FUNCTION_BLOCK FB_IEDClient IMPLEMENTS I_ScsmAbortIndEventSink, I_ScsmGetServerDirectoryCnfEventSink, I_ScsmGetLogicalDeviceDirectoryCnfEventSink, I_ScsmGetLogicalNodeDirectoryCnfEventSink, I_ScsmGetDataValuesCnfEventSink, I_ScsmSetDataValuesCnfEventSink, I_ScsmReportIndEventSink, I_ScsmControlCnfEventSink, I_ScsmLastApplErrorIndEventSink, I_ScsmCommandTerminationIndEventSink
VAR_INPUT
	fbConnection		: FB_iec61850ClientClass := (ipAbortInd:=THIS^, ipGetServerDirectoryCnf:=THIS^, ipGetLogicalDeviceDirectoryCnf:=THIS^, ipGetLogicalNodeDirectoryCnf:=THIS^, ipGetDataValuesCnf:=THIS^, ipSetDataValuesCnf:=THIS^, ipReportInd:=THIS^, ipControlCnf:=THIS^, ipLastApplErrorInd:=THIS^, ipCommandTerminationInd:=THIS^);
END_VAR
VAR
	_bAbort				: BOOL; (* Rising edge activates AbortReq() command execution *)
	_bDisconnect		: BOOL; (* Rising edge activates ReleaseReq() command execution *)
	_bConnect			: BOOL; (* Rising edge activates AssociateReq() command execution *)
	_bReconnect			: BOOL := TRUE; (* TRUE => reconnect automatically *)
	_bReadAllData		: BOOL := TRUE; (* TRUE => read/refresh all data values on reconnect *)
	
	state				: BYTE;
	eState				: E_AsyncEnvironmentState; (* Environment state *)
	bBusy				: BOOL; (* If TRUE => command execution is busy *)
	bSuccess			: BOOL;
	ipResult			: I_AsyncServiceResultClass;
	sLastErrorResult	: T_MaxString;
	fbAbortReason		: FB_ServiceErrorClass := (stError:=SUCCESS_EVENT);
	sLastAbortReason	: T_MaxString;
	nInvokeID			: UDINT;
	eServiceError		: E_AcsiServiceError; (* Latest OnXyzCnf() or OnXyzInd() event handler error *)
	nServiceError		: UDINT; (* Counts OnXyzCnf() and OnXyzInd() event handler errors *)
	nCmdError			: UDINT; (* Counts xyzReq() command errors *)
	sObjReference		: T_AcsiObjectReference; (* DATA object reference *)
	sCtrlReference		: T_AcsiObjectReference; (* CONTROLLABLE-DATA object reference *)

	bGetServerDirectory				: BOOL := TRUE; (* Rising edge enumerates logical-devices *)
	bGetLogicalDeviceDirectory		: BOOL := TRUE; (* Rising edge enumerates logical-nodes *)
	bGetLogicalNodeDirectory		: BOOL := TRUE; (* Rising edge enumerates "IEDLD1/LLN0" data-sets *)
	bGetAllServerValues				: BOOL := TRUE; (* Rising edge reads all "IEDLD1" data attribute values *)
	bGetAllDataValues_LLN0_ST		: BOOL := TRUE; (* Rising edge reads all "IEDLD1/LLN0.ST" data attribute values (having selected functional constraint) *)
	bGetDataValues_LLN0_ST_Beh		: BOOL := TRUE; (* Rising edge reads all "IEDLD1/LLN0.ST.Beh" data attribute values (having selected functional constraint) *)

	(* Low-Level/basic control of reporting using single commands to read/write RCB data attribute values *)
	bGetUrCBValues_urcb101			: BOOL := TRUE; (* Rising edge reads all "IEDLD1/LLN0.urcb101" data attribute values *)
	bGetUrCBValues_urcb201			: BOOL := TRUE; (* Rising edge reads all "IEDLD1/LLN0.urcb201" data attribute values *)
	bGetUrCBValues_urcb301			: BOOL := TRUE; (* Rising edge reads all "IEDLD1/LLN0.urcb301" data attribute values *)
	bGetBrCBValues_brcb101			: BOOL := TRUE; (* Rising edge reads all "IEDLD1/LLN0.brcb101" data attribute values *)
	bGetBrCBValues_brcb201			: BOOL := TRUE; (* Rising edge reads all "IEDLD1/LLN0.brcb201" data attribute values *)
	bGetBrCBValues_brcb301			: BOOL := TRUE; (* Rising edge reads all "IEDLD1/LLN0.brcb301" data attribute values *)

	eSetUrCBValues_urcb101_Resv		: E_CtlBool := E_CtlBool.None; (* Writes True|False to "IEDLD1/LLN0.urcb101.Resv" data attribute value *)
	eSetUrCBValues_urcb101_RptEna	: E_CtlBool := E_CtlBool.None; (* Writes True|False to "IEDLD1/LLN0.urcb101.RptEna" data attribute value *)
	bSetUrCBValues_urcb101_RptID	: BOOL := FALSE; (* Rising edge writes "IEDLD1/LLN0.urcb101.RptID" data attribute value *)
	bSetUrCBValues_urcb101_TrgOps	: BOOL := FALSE; (* Rising edge writes "IEDLD1/LLN0.urcb101.TrgOps" data attribute value *)
	bSetUrCBValues_urcb101_OptFlds	: BOOL := FALSE; (* Rising edge writes "IEDLD1/LLN0.urcb101.OptFlds" data attribute value *)
	bSetUrCBValues_urcb101_IntgPd	: BOOL := FALSE; (* Rising edge writes "IEDLD1/LLN0.urcb101.IntgPd" data attribute value *)
	bSetUrCBValues_urcb101_BufTm	: BOOL := FALSE; (* Rising edge writes "IEDLD1/LLN0.urcb101.BufTm" data attribute value *)
	bSetUrCBValues_urcb101_All		: BOOL := FALSE; (* Rising edge writes multiple "IEDLD1/LLN0.urcb101" data attribute values: "RptID", "TrgOps", "OptFlds, "IntgPd" and "BufTm" *)

	eSetBrCBValues_brcb101_RptEna	: E_CtlBool := E_CtlBool.None; (* Writes True|False to "IEDLD1/LLN0.brcb101.RptEna" data attribute value *)
	bSetBrCBValues_brcb101_RptID	: BOOL := FALSE; (* Rising edge writes "IEDLD1/LLN0.brcb101.RptID" data attribute value *)
	bSetBrCBValues_brcb101_TrgOps	: BOOL := FALSE; (* Rising edge writes "IEDLD1/LLN0.brcb101.TrgOps" data attribute value *)
	bSetBrCBValues_brcb101_OptFlds	: BOOL := FALSE; (* Rising edge writes "IEDLD1/LLN0.brcb101.OptFlds" data attribute value *)
	bSetBrCBValues_brcb101_IntgPd	: BOOL := FALSE; (* Rising edge writes "IEDLD1/LLN0.brcb101.IntgPd" data attribute value *)
	bSetBrCBValues_brcb101_BufTm	: BOOL := FALSE; (* Rising edge writes "IEDLD1/LLN0.brcb101.BufTm" data attribute value *)
	bSetBrCBValues_brcb101_All		: BOOL := FALSE; (* Rising edge writes multiple "IEDLD1/LLN0.brcb101" data attribute values: "RptID", "TrgOps", "OptFlds", "IntgPd" and "BufTm" *)

	(* High-Level control of reporting using "Client" function block instances attached to RCB *)
	eControl_IEDLD1_LLN0_urcb101	: E_AcsiCtlReport := E_AcsiCtlReport.None; (* Control unbuffered reports using "IEDLD1/LLN0.urcb101.Client" function block, Enable|Disable|GI *)
	eControl_IEDLD1_LLN0_urcb201	: E_AcsiCtlReport := E_AcsiCtlReport.None; (* Control unbuffered reports using "IEDLD1/LLN0.urcb201.Client" function block, Enable|Disable|GI *)
	eControl_IEDLD1_LLN0_urcb301	: E_AcsiCtlReport := E_AcsiCtlReport.None; (* Control unbuffered reports using "IEDLD1/LLN0.urcb301.Client" function block, Enable|Disable|GI *)
	eControl_IEDLD1_LLN0_brcb101	: E_AcsiCtlReport := E_AcsiCtlReport.None; (* Control buffered reports using "IEDLD1/LLN0.brcb101.Client" function block, Enable|Disable|GI|PurgeBuf/Resync *)
	eControl_IEDLD1_LLN0_brcb201	: E_AcsiCtlReport := E_AcsiCtlReport.None; (* Control buffered reports using "IEDLD1/LLN0.brcb201.Client" function block, Enable|Disable|GI|PurgeBuf/Resync *)
	eControl_IEDLD1_LLN0_brcb301	: E_AcsiCtlReport := E_AcsiCtlReport.None; (* Control buffered reports using "IEDLD1/LLN0.brcb301.Client" function block, Enable|Disable|GI|PurgeBuf/Resync *)

	(* Some temporary variables used to configure the report behaviour *)
	stSet_urcb						: ST_ScsmUrCBValuesSet;(* URCB selection flags used by SetUrCBValuesReq() command *)
	stSet_brcb						: ST_ScsmBrCBValuesSet;(* BRCB selection flags use by SetBrCBValuesReq() command *)
	usrTrgOps						: ST_AcsiTriggerConditions;(* User defined "TrgOps" data attribute value *)
	usrOptFlds						: ST_AcsiOptionalFields;(* User defined "OptFlds" data attribute value *)

	Last_Rx_brcb101_nEntryID		: LWORD;(* Last received buffered report EntryID *)
	Last_Rx_brcb201_nEntryID		: LWORD;(* Last received buffered report EntryID *)
	Last_Rx_brcb301_nEntryID		: LWORD;(* Last received buffered report EntryID *)
END_VAR

fbConnection.Execute();
eState:= fbConnection.eState;

CASE state OF
	0: (* Initial state *)
		IF _bAbort THEN (* Abort connection => execute AbortReq() command *)
			_bAbort:= FALSE;
			bSuccess:= fbConnection.AbortReq(ipReason:=fbAbortReason, ipSink:=0, ipResult=>ipResult);
			state:= SEL(bSuccess, 100, 1);
		ELSIF eState = E_AsyncEnvironmentState.Idle AND (_bConnect OR _bReconnect) THEN (* Open/establish connection => execute AssociateReq() command *)
			_bConnect:= FALSE;
			bGetAllServerValues:= SEL(_bReadAllData, bGetAllServerValues, TRUE);
			bSuccess:= fbConnection.AssociateReq(ipSink:=0, ipResult=>ipResult);
			state:= SEL(bSuccess, 100, 1);
		ELSIF eState = E_AsyncEnvironmentState.Established AND _bDisconnect THEN (* Close/release connection => execute ReleaseReq() command *)
			_bDisconnect:= FALSE;
			bSuccess:= fbConnection.ReleaseReq(ipSink:=0, ipResult=>ipResult);
			state:= SEL(bSuccess, 100, 1);
		ELSIF eState = E_AsyncEnvironmentState.Established THEN (* Connection established => exchange IED data *)
			state:= 10;
		END_IF
		_bConnect:= FALSE;
		_bDisconnect:= FALSE;
		(*==================================================================================================================================================================*)
	1: (* Wait for AbortReq() or ReleaseReq() or AssociateReq() command completion *)
		IF ipResult <> 0 THEN
			ipResult.Execute();
			IF NOT (bBusy:=ipResult.IsBusy()) THEN
				state:= SEL(ipResult.IsCompleted(), 100(* failed or aborted *), 0(* succeeded *));
			END_IF
		END_IF
		(*==================================================================================================================================================================*)
	10: (* Read/Write IED data *)
		IF bGetServerDirectory THEN (* Example => execute GetServerDirectoryReq() command *)
			bGetServerDirectory:= FALSE;
			bSuccess:= fbConnection.GetServerDirectoryReq(ipServer:=fbIED, eClass:=E_AcsiServerDirectoryClass.LogicalDevice, hUser:=0, ipSink:=0, nInvokeID=>nInvokeID, ipResult=>ipResult);
			state:= SEL(bSuccess, 100, 11);
		ELSIF bGetLogicalDeviceDirectory THEN (* Example => execute GetLogicalDeviceDirectoryReq() command *)
			bGetLogicalDeviceDirectory:= FALSE;
			bSuccess:= fbConnection.GetLogicalDeviceDirectoryReq(ipLogicalDevice:=fbIED.IEDLD1, hUser:=0, ipSink:=0, nInvokeID=>nInvokeID, ipResult=>ipResult);
			state:= SEL(bSuccess, 100, 11);
		ELSIF bGetLogicalNodeDirectory THEN (* Example => execute GetLogicalNodeDirectoryReq() command *)
			bGetLogicalNodeDirectory:= FALSE;
			bSuccess:= fbConnection.GetLogicalNodeDirectoryReq(ipLogicalNode:=fbIED.IEDLD1.LLN0, eClass:=E_AcsiLogicalNodeClass.DataSet, hUser:=0, ipSink:=0, nInvokeID=>nInvokeID, ipResult=>ipResult);
			state:= SEL(bSuccess, 100, 11);
		ELSIF bGetAllServerValues THEN (* Example => execute GetAllServerValues() command *)
			bGetAllServerValues:= FALSE;
			bSuccess:= fbConnection.GetAllServerValuesReq(ipServer:=fbIED, hUser:=0, ipSink:=0, nInvokeID=>nInvokeID, ipResult=>ipResult);
			state:= SEL(bSuccess, 100, 11);
		ELSIF bGetAllDataValues_LLN0_ST THEN (* Example => execute GetAllDataValuesReq() command *)
			bGetAllDataValues_LLN0_ST:= FALSE;
			bSuccess:= fbConnection.GetAllDataValuesReq(ipLogicalNode:=fbIED.IEDLD1.LLN0, eFc:=E_AcsiFc.ST_, hUser:=0, ipSink:=0, nInvokeID=>nInvokeID, ipResult=>ipResult);
			state:= SEL(bSuccess, 100, 11);
		ELSIF bGetDataValues_LLN0_ST_Beh THEN (* Example => execute GetDataValuesReq() command *)
			bGetDataValues_LLN0_ST_Beh:= FALSE;
			bSuccess:= fbConnection.GetDataValuesReq(ipData:=fbIED.IEDLD1.LLN0.Beh, eFc:=E_AcsiFc.ST_, hUser:=0, ipSink:=0, nInvokeID=>nInvokeID, ipResult=>ipResult);
			state:= SEL(bSuccess, 100, 11);
	
		(*==================================================================================================================================================================*)
		(*                        Low-Level/basic control of reporting using single commands to read/write RCB data attribute values                                        *)
		(*==================================================================================================================================================================*)
		
		(* Read all "IEDLD1/LLN0.urcb101" data attribute values *)
		ELSIF bGetUrCBValues_urcb101 THEN (* Example => execute GetUrCBValuesReq() command *)
			bGetUrCBValues_urcb101:= FALSE; (* Reset flag to recognize next rising edge *)
			bSuccess:= fbConnection.GetUrCBValuesReq(ipUrCB:=fbIED.IEDLD1.LLN0.urcb101, hUser:=0, ipSink:=0, nInvokeID=>nInvokeID, ipResult=>ipResult); (* Activation of command execution *)
			state:= SEL(bSuccess, 100, 11); (* If command activation succeeded then wait for command completion else report an error *)

		(* Read all "IEDLD1/LLN0.urcb201" data attribute values *)
		ELSIF bGetUrCBValues_urcb201 THEN (* Example => execute GetUrCBValuesReq() command *)
			bGetUrCBValues_urcb201:= FALSE; (* Reset flag to recognize next rising edge *)
			bSuccess:= fbConnection.GetUrCBValuesReq(ipUrCB:=fbIED.IEDLD1.LLN0.urcb201, hUser:=0, ipSink:=0, nInvokeID=>nInvokeID, ipResult=>ipResult); (* Activation of command execution *)
			state:= SEL(bSuccess, 100, 11); (* If command activation succeeded then wait for command completion else report an error *)

		(* Read all "IEDLD1/LLN0.urcb301" data attribute values *)
		ELSIF bGetUrCBValues_urcb301 THEN (* Example => execute GetUrCBValuesReq() command *)
			bGetUrCBValues_urcb301:= FALSE; (* Reset flag to recognize next rising edge *)
			bSuccess:= fbConnection.GetUrCBValuesReq(ipUrCB:=fbIED.IEDLD1.LLN0.urcb301, hUser:=0, ipSink:=0, nInvokeID=>nInvokeID, ipResult=>ipResult); (* Activation of command execution *)
			state:= SEL(bSuccess, 100, 11); (* If command activation succeeded then wait for command completion else report an error *)

		(*==================================================================================================================================================================*)
		(* Read all "IEDLD1/LLN0.brcb101" data attribute values *)
		ELSIF bGetBrCBValues_brcb101 THEN (* Example => execute GetBrCBValuesReq() command *)
			bGetBrCBValues_brcb101:= FALSE; (* Reset flag to recognize next rising edge *)
			bSuccess:= fbConnection.GetBrCBValuesReq(ipBrCB:=fbIED.IEDLD1.LLN0.brcb101, hUser:=0, ipSink:=0, nInvokeID=>nInvokeID, ipResult=>ipResult); (* Activation of command execution *)
			state:= SEL(bSuccess, 100, 11); (* If command activation succeeded then wait for command completion else report an error *)

		(* Read all "IEDLD1/LLN0.brcb201" data attribute values *)
		ELSIF bGetBrCBValues_brcb201 THEN (* Example => execute GetBrCBValuesReq() command *)
			bGetBrCBValues_brcb201:= FALSE; (* Reset flag to recognize next rising edge *)
			bSuccess:= fbConnection.GetBrCBValuesReq(ipBrCB:=fbIED.IEDLD1.LLN0.brcb201, hUser:=0, ipSink:=0, nInvokeID=>nInvokeID, ipResult=>ipResult); (* Activation of command execution *)
			state:= SEL(bSuccess, 100, 11); (* If command activation succeeded then wait for command completion else report an error *)

		(* Read all "IEDLD1/LLN0.brcb301" data attribute values *)
		ELSIF bGetBrCBValues_brcb301 THEN (* Example => execute GetBrCBValuesReq() command *)
			bGetBrCBValues_brcb301:= FALSE; (* Reset flag to recognize next rising edge *)
			bSuccess:= fbConnection.GetBrCBValuesReq(ipBrCB:=fbIED.IEDLD1.LLN0.brcb301, hUser:=0, ipSink:=0, nInvokeID=>nInvokeID, ipResult=>ipResult); (* Activation of command execution *)
			state:= SEL(bSuccess, 100, 11); (* If command activation succeeded then wait for command completion else report an error *)

		(*==================================================================================================================================================================*)
		(* Write "IEDLD1/LLN0.urcb101.RptID" data attribute value *)
		ELSIF bSetUrCBValues_urcb101_RptID THEN (* Example => execute SetUrCBValuesReq() command *)
			bSetUrCBValues_urcb101_RptID:= FALSE; (* Reset flag to recognize next rising edge *)
			memset(ADR(stSet_urcb), 0, SIZEOF(stSet_urcb)); (* Clear all URCB attribute selection flags *)
			stSet_urcb.RptID:= TRUE; (* Select URCB->RptID attribute to be written *)
			fbIED.IEDLD1.LLN0.urcb101.RptID.sValue:= fbIED.IEDLD1.LLN0.urcb101.RptID.sConfig; (* Set new data attribute value to be written *)
			bSuccess:= fbConnection.SetUrCBValuesReq(ipUrCB:=fbIED.IEDLD1.LLN0.urcb101, stSet:=stSet_urcb, hUser:=0, ipSink:=0, nInvokeID=>nInvokeID, ipResult=>ipResult); (* Activation of command execution *)
			state:= SEL(bSuccess, 100, 11); (* If command activation succeeded then wait for command completion else report an error *)

		(*==================================================================================================================================================================*)
		(* Write "IEDLD1/LLN0.urcb101.TrgOps" data attribute value *)
		ELSIF bSetUrCBValues_urcb101_TrgOps THEN (* Example => execute SetUrCBValuesReq() command *)
			bSetUrCBValues_urcb101_TrgOps:= FALSE; (* Reset flag to recognize next rising edge *)
			memset(ADR(stSet_urcb), 0, SIZEOF(stSet_urcb)); (* Clear all URCB attribute selection flags *)
			stSet_urcb.TrgOps:= TRUE; (* Select URCB->TrgOps attribute to be written *)
			fbIED.IEDLD1.LLN0.urcb101.TrgOps.cValue:= fbIED.IEDLD1.LLN0.urcb101.TrgOps.cConfig; (* Set new data attribute value to be written *)
			bSuccess:= fbConnection.SetUrCBValuesReq(ipUrCB:=fbIED.IEDLD1.LLN0.urcb101, stSet:=stSet_urcb, hUser:=0, ipSink:=0, nInvokeID=>nInvokeID, ipResult=>ipResult); (* Activation of command execution *)
			state:= SEL(bSuccess, 100, 11); (* If command activation succeeded then wait for command completion else report an error *)

		(*==================================================================================================================================================================*)
		(* Write "IEDLD1/LLN0.urcb101.OptFlds" data attribute value *)
		ELSIF bSetUrCBValues_urcb101_OptFlds THEN (* Example => execute SetUrCBValuesReq() command *)
			bSetUrCBValues_urcb101_OptFlds:= FALSE; (* Reset flag to recognize next rising edge *)
			memset(ADR(stSet_urcb), 0, SIZEOF(stSet_urcb)); (* Clear all URCB attribute selection flags *)
			stSet_urcb.OptFlds:= TRUE; (* Select URCB->OptFlds attribute to be written *)
			fbIED.IEDLD1.LLN0.urcb101.OptFlds.cValue:= fbIED.IEDLD1.LLN0.urcb101.OptFlds.cValue; (* Set new data attribute value to be written *)
			bSuccess:= fbConnection.SetUrCBValuesReq(ipUrCB:=fbIED.IEDLD1.LLN0.urcb101, stSet:=stSet_urcb, hUser:=0, ipSink:=0, nInvokeID=>nInvokeID, ipResult=>ipResult); (* Activation of command execution *)
			state:= SEL(bSuccess, 100, 11); (* If command activation succeeded then wait for command completion else report an error *)

		(*==================================================================================================================================================================*)
		(* Write "IEDLD1/LLN0.urcb101.IntgPd" data attribute value *)
		ELSIF bSetUrCBValues_urcb101_IntgPd THEN (* Example => execute SetUrCBValuesReq() command *)
			bSetUrCBValues_urcb101_IntgPd:= FALSE; (* Reset flag to recognize next rising edge *)
			memset(ADR(stSet_urcb), 0, SIZEOF(stSet_urcb)); (* Clear all URCB attribute selection flags *)
			stSet_urcb.IntgPd:= TRUE; (* Select URCB->IntgPd attribute to be written *)
			fbIED.IEDLD1.LLN0.urcb101.IntgPd.nValue:= fbIED.IEDLD1.LLN0.urcb101.IntgPd.nConfig; (* Set new data attribute value to be written *)
			bSuccess:= fbConnection.SetUrCBValuesReq(ipUrCB:=fbIED.IEDLD1.LLN0.urcb101, stSet:=stSet_urcb, hUser:=0, ipSink:=0, nInvokeID=>nInvokeID, ipResult=>ipResult); (* Activation of command execution *)
			state:= SEL(bSuccess, 100, 11); (* If command activation succeeded then wait for command completion else report an error *)

		(*==================================================================================================================================================================*)
		(* Write "IEDLD1/LLN0.urcb101.BufTm" data attribute value *)
		ELSIF bSetUrCBValues_urcb101_BufTm THEN (* Example => execute SetUrCBValuesReq() command *)
			bSetUrCBValues_urcb101_BufTm:= FALSE; (* Reset flag to recognize next rising edge *)
			memset(ADR(stSet_urcb), 0, SIZEOF(stSet_urcb)); (* Clear all URCB attribute selection flags *)
			stSet_urcb.BufTm:= TRUE; (* Select URCB->BufTm attribute to be written *)
			fbIED.IEDLD1.LLN0.urcb101.BufTm.nValue:= fbIED.IEDLD1.LLN0.urcb101.BufTm.nConfig; (* Set new data attribute value to be written *)
			bSuccess:= fbConnection.SetUrCBValuesReq(ipUrCB:=fbIED.IEDLD1.LLN0.urcb101, stSet:=stSet_urcb, hUser:=0, ipSink:=0, nInvokeID=>nInvokeID, ipResult=>ipResult); (* Activation of command execution *)
			state:= SEL(bSuccess, 100, 11); (* If command activation succeeded then wait for command completion else report an error *)

		(*==================================================================================================================================================================*)
		(* Write multiple "IEDLD1/LLN0.urcb101" data attribute values: "RptID", "TrgOps", "OptFlds", "IntgPd" and "BufTm" *)
		ELSIF bSetUrCBValues_urcb101_All THEN (* Example => execute SetUrCBValuesReq() command *)
			bSetUrCBValues_urcb101_All:= FALSE; (* Reset flag to recognize next rising edge *)
			memset(ADR(stSet_urcb), 0, SIZEOF(stSet_urcb)); (* Clear all URCB attribute selection flags *)
			stSet_urcb.RptID:= TRUE; (* Select URCB->RptID attribute to be written *)
			stSet_urcb.TrgOps:= TRUE; (* Select URCB->TrgOps attribute to be written *)
			stSet_urcb.OptFlds:= TRUE; (* Select URCB->OptFlds attribute to be written *)
			stSet_urcb.IntgPd:= TRUE; (* Select URCB->IntgPd attribute to be written *)
			stSet_urcb.BufTm:= TRUE; (* Select URCB->BufTm attribute to be written *)
			fbIED.IEDLD1.LLN0.urcb101.RptID.sValue:= fbIED.IEDLD1.LLN0.urcb101.RptID.sConfig; (* Set new "RptID" data attribute value to be written *)
			fbIED.IEDLD1.LLN0.urcb101.TrgOps.cValue:= fbIED.IEDLD1.LLN0.urcb101.TrgOps.cConfig; (* Set new "TrgOps" data attribute value to be written *)
			fbIED.IEDLD1.LLN0.urcb101.OptFlds.cValue:= fbIED.IEDLD1.LLN0.urcb101.OptFlds.cConfig; (* Set new "OptFlds" data attribute value to be written *)
			fbIED.IEDLD1.LLN0.urcb101.IntgPd.nValue:= fbIED.IEDLD1.LLN0.urcb101.IntgPd.nConfig; (* Set new "IntgPd" data attribute value to be written *)
			fbIED.IEDLD1.LLN0.urcb101.BufTm.nValue:= fbIED.IEDLD1.LLN0.urcb101.BufTm.nConfig; (* Set new "BufTm" data attribute value to be written *)
			bSuccess:= fbConnection.SetUrCBValuesReq(ipUrCB:=fbIED.IEDLD1.LLN0.urcb101, stSet:=stSet_urcb, hUser:=0, ipSink:=0, nInvokeID=>nInvokeID, ipResult=>ipResult); (* Activation of command execution *)
			state:= SEL(bSuccess, 100, 11); (* If command activation succeeded then wait for command completion else report an error *)

		(*==================================================================================================================================================================*)
		(* Write "IEDLD1/LLN0.urcb101.Resv" data attribute value: True|False *)
		ELSIF eSetUrCBValues_urcb101_Resv <> E_CtlBool.None THEN (* Example => execute SetUrCBValuesReq() command *)
			memset(ADR(stSet_urcb), 0, SIZEOF(stSet_urcb)); (* Clear all URCB attribute selection flags *)
			stSet_urcb.Resv:= TRUE; (* Select URCB->Resv attribute to be written *)
			fbIED.IEDLD1.LLN0.urcb101.Resv.bValue:= SEL(eSetUrCBValues_urcb101_Resv = E_CtlBool.Enable, FALSE, TRUE); (* Set new data attribute value to be written *)
			bSuccess:= fbConnection.SetUrCBValuesReq(ipUrCB:=fbIED.IEDLD1.LLN0.urcb101, stSet:=stSet_urcb, hUser:=0, ipSink:=0, nInvokeID=>nInvokeID, ipResult=>ipResult); (* Activation of command execution *)
			state:= SEL(bSuccess, 100, 11); (* If command activation succeeded then wait for command completion else report an error *)
			eSetUrCBValues_urcb101_Resv:= E_CtlBool.None; (* Reset enum value to recognize next write request *)

		(*==================================================================================================================================================================*)
		(* Write "IEDLD1/LLN0.urcb101.RptEna" data attribute value: True|False *)
		ELSIF eSetUrCBValues_urcb101_RptEna <> E_CtlBool.None THEN (* Example => execute SetUrCBValuesReq() command *)
			memset(ADR(stSet_urcb), 0, SIZEOF(stSet_urcb)); (* Clear all URCB attribute selection flags *)
			stSet_urcb.RptEna:= TRUE; (* Select URCB->RptEna attribute to be written *)
			fbIED.IEDLD1.LLN0.urcb101.RptEna.bValue:= SEL(eSetUrCBValues_urcb101_RptEna = E_CtlBool.Enable, FALSE, TRUE); (* Set new data attribute value to be written *)
			bSuccess:= fbConnection.SetUrCBValuesReq(ipUrCB:=fbIED.IEDLD1.LLN0.urcb101, stSet:=stSet_urcb, hUser:=0, ipSink:=0, nInvokeID=>nInvokeID, ipResult=>ipResult); (* Activation of command execution *)
			state:= SEL(bSuccess, 100, 11); (* If command activation succeeded then wait for command completion else report an error *)
			eSetUrCBValues_urcb101_RptEna:= E_CtlBool.None; (* Reset enum value to recognize next write request *)

		(*==================================================================================================================================================================*)
		(* Write "IEDLD1/LLN0.brcb101.RptID" data attribute value *)
		ELSIF bSetBrCBValues_brcb101_RptID THEN (* Example => execute SetBrCBValuesReq() command *)
			bSetBrCBValues_brcb101_RptID:= FALSE; (* Reset flag to recognize next rising edge *)
			memset(ADR(stSet_brcb), 0, SIZEOF(stSet_brcb)); (* Clear all BRCB attribute selection flags *)
			stSet_brcb.RptID:= TRUE; (* Select BRCB->RptID attribute to be written *)
			fbIED.IEDLD1.LLN0.brcb101.RptID.sValue:= fbIED.IEDLD1.LLN0.brcb101.RptID.sConfig; (* Set new data attribute value to be written *)
			bSuccess:= fbConnection.SetBrCBValuesReq(ipBrCB:=fbIED.IEDLD1.LLN0.brcb101, stSet:=stSet_brcb, hUser:=0, ipSink:=0, nInvokeID=>nInvokeID, ipResult=>ipResult); (* Activation of command execution *)
			state:= SEL(bSuccess, 100, 11); (* If command activation succeeded then wait for command completion else report an error *)

		(*==================================================================================================================================================================*)
		(* Write "IEDLD1/LLN0.brcb101.TrgOps" data attribute value *)
		ELSIF bSetBrCBValues_brcb101_TrgOps THEN (* Example => execute SetBrCBValuesReq() command *)
			bSetBrCBValues_brcb101_TrgOps:= FALSE; (* Reset flag to recognize next rising edge *)
			memset(ADR(stSet_brcb), 0, SIZEOF(stSet_brcb)); (* Clear all BRCB attribute selection flags *)
			stSet_brcb.TrgOps:= TRUE; (* Select BRCB->TrgOps attribute to be written *)
			fbIED.IEDLD1.LLN0.brcb101.TrgOps.cValue:= fbIED.IEDLD1.LLN0.brcb101.TrgOps.cConfig; (* Set new data attribute value to be written *)
			bSuccess:= fbConnection.SetBrCBValuesReq(ipBrCB:=fbIED.IEDLD1.LLN0.brcb101, stSet:=stSet_brcb, hUser:=0, ipSink:=0, nInvokeID=>nInvokeID, ipResult=>ipResult); (* Activation of command execution *)
			state:= SEL(bSuccess, 100, 11); (* If command activation succeeded then wait for command completion else report an error *)

		(*==================================================================================================================================================================*)
		(* Write "IEDLD1/LLN0.brcb101.OptFlds" data attribute value *)
		ELSIF bSetBrCBValues_brcb101_OptFlds THEN (* Example => execute SetBrCBValuesReq() command *)
			bSetBrCBValues_brcb101_OptFlds:= FALSE; (* Reset flag to recognize next rising edge *)
			memset(ADR(stSet_brcb), 0, SIZEOF(stSet_brcb)); (* Clear all BRCB attribute selection flags *)
			stSet_brcb.OptFlds:= TRUE; (* Select BRCB->OptFlds attribute to be written *)
			fbIED.IEDLD1.LLN0.brcb101.OptFlds.cValue:= fbIED.IEDLD1.LLN0.brcb101.OptFlds.cValue; (* Set new data attribute value to be written *)
			bSuccess:= fbConnection.SetBrCBValuesReq(ipBrCB:=fbIED.IEDLD1.LLN0.brcb101, stSet:=stSet_brcb, hUser:=0, ipSink:=0, nInvokeID=>nInvokeID, ipResult=>ipResult); (* Activation of command execution *)
			state:= SEL(bSuccess, 100, 11); (* If command activation succeeded then wait for command completion else report an error *)

		(*==================================================================================================================================================================*)
		(* Write "IEDLD1/LLN0.brcb101.IntgPd" data attribute value *)
		ELSIF bSetBrCBValues_brcb101_IntgPd THEN (* Example => execute SetBrCBValuesReq() command *)
			bSetBrCBValues_brcb101_IntgPd:= FALSE; (* Reset flag to recognize next rising edge *)
			memset(ADR(stSet_brcb), 0, SIZEOF(stSet_brcb)); (* Clear all BRCB attribute selection flags *)
			stSet_brcb.IntgPd:= TRUE; (* Select BRCB->IntgPd attribute to be written *)
			fbIED.IEDLD1.LLN0.brcb101.IntgPd.nValue:= fbIED.IEDLD1.LLN0.brcb101.IntgPd.nConfig; (* Set new data attribute value to be written *)
			bSuccess:= fbConnection.SetBrCBValuesReq(ipBrCB:=fbIED.IEDLD1.LLN0.brcb101, stSet:=stSet_brcb, hUser:=0, ipSink:=0, nInvokeID=>nInvokeID, ipResult=>ipResult); (* Activation of command execution *)
			state:= SEL(bSuccess, 100, 11); (* If command activation succeeded then wait for command completion else report an error *)

		(*==================================================================================================================================================================*)
		(* Write "IEDLD1/LLN0.brcb101.BufTm" data attribute value *)
		ELSIF bSetBrCBValues_brcb101_BufTm THEN (* Example => execute SetBrCBValuesReq() command *)
			bSetBrCBValues_brcb101_BufTm:= FALSE; (* Reset flag to recognize next rising edge *)
			memset(ADR(stSet_brcb), 0, SIZEOF(stSet_brcb)); (* Clear all BRCB attribute selection flags *)
			stSet_brcb.BufTm:= TRUE; (* Select BRCB->BufTm attribute to be written *)
			fbIED.IEDLD1.LLN0.brcb101.BufTm.nValue:= fbIED.IEDLD1.LLN0.brcb101.BufTm.nConfig; (* Set new data attribute value to be written *)
			bSuccess:= fbConnection.SetBrCBValuesReq(ipBrCB:=fbIED.IEDLD1.LLN0.brcb101, stSet:=stSet_brcb, hUser:=0, ipSink:=0, nInvokeID=>nInvokeID, ipResult=>ipResult); (* Activation of command execution *)
			state:= SEL(bSuccess, 100, 11); (* If command activation succeeded then wait for command completion else report an error *)

		(*==================================================================================================================================================================*)
		(* Write multiple "IEDLD1/LLN0.brcb101" data attribute values: "TrgOps", "OptFlds", "IntgPd" and "BufTm" *)
		ELSIF bSetBrCBValues_brcb101_All THEN (* Example => execute SetBrCBValuesReq() command *)
			bSetBrCBValues_brcb101_All:= FALSE; (* Reset flag to recognize next rising edge *)
			memset(ADR(stSet_brcb), 0, SIZEOF(stSet_brcb)); (* Clear all BRCB attribute selection flags *)
			stSet_brcb.RptID:= TRUE; (* Select BRCB->RptID attribute to be written *)
			stSet_brcb.TrgOps:= TRUE; (* Select BRCB->TrgOps attribute to be written *)
			stSet_brcb.OptFlds:= TRUE; (* Select BRCB->OptFlds attribute to be written *)
			stSet_brcb.IntgPd:= TRUE; (* Select BRCB->IntgPd attribute to be written *)
			stSet_brcb.BufTm:= TRUE; (* Select BRCB->BufTm attribute to be written *)
			fbIED.IEDLD1.LLN0.brcb101.RptID.sValue:= fbIED.IEDLD1.LLN0.brcb101.RptID.sConfig; (* Set new "RptID" data attribute value to be written *)
			fbIED.IEDLD1.LLN0.brcb101.TrgOps.cValue:= fbIED.IEDLD1.LLN0.brcb101.TrgOps.cConfig; (* Set new "TrgOps" data attribute value to be written *)
			fbIED.IEDLD1.LLN0.brcb101.OptFlds.cValue:= fbIED.IEDLD1.LLN0.brcb101.OptFlds.cConfig; (* Set new "OptFlds" data attribute value to be written *)
			fbIED.IEDLD1.LLN0.brcb101.IntgPd.nValue:= fbIED.IEDLD1.LLN0.brcb101.IntgPd.nConfig; (* Set new "IntgPd" data attribute value to be written *)
			fbIED.IEDLD1.LLN0.brcb101.BufTm.nValue:= fbIED.IEDLD1.LLN0.brcb101.BufTm.nConfig; (* Set new "BufTm" data attribute value to be written *)
			bSuccess:= fbConnection.SetBrCBValuesReq(ipBrCB:=fbIED.IEDLD1.LLN0.brcb101, stSet:=stSet_brcb, hUser:=0, ipSink:=0, nInvokeID=>nInvokeID, ipResult=>ipResult); (* Activation of command execution *)
			state:= SEL(bSuccess, 100, 11); (* If command activation succeeded then wait for command completion else report an error *)

		(*==================================================================================================================================================================*)
		(* Write "IEDLD1/LLN0.brcb101.RptEna" data attribute value *)
		ELSIF eSetBrCBValues_brcb101_RptEna <> E_CtlBool.None THEN (* Example => execute SetBrCBValuesReq() command *)
			memset(ADR(stSet_brcb), 0, SIZEOF(stSet_brcb)); (* Clear all BRCB attribute selection flags *)
			stSet_brcb.RptEna:= TRUE; (* Select BRCB->RptEna attribute to be written *)
			fbIED.IEDLD1.LLN0.brcb101.RptEna.bValue:= SEL(eSetBrCBValues_brcb101_RptEna = E_CtlBool.Enable, FALSE, TRUE); (* Set new data attribute value to be written *)
			bSuccess:= fbConnection.SetBrCBValuesReq(ipBrCB:=fbIED.IEDLD1.LLN0.brcb101, stSet:=stSet_brcb, hUser:=0, ipSink:=0, nInvokeID=>nInvokeID, ipResult=>ipResult); (* Activation of command execution *)
			state:= SEL(bSuccess, 100, 11); (* If command activation succeeded then wait for command completion else report an error *)
			eSetBrCBValues_brcb101_RptEna:= E_CtlBool.None; (* Reset enum value to recognize next write request *)

		(*==================================================================================================================================================================*)
		(*                            High-Level control of reporting using "Client" function block instances attached to RCB                                               *)
		
		(*==================================================================================================================================================================*)
		(* Control unbuffered reports using "IEDLD1/LLN0.urcb101.Client" function block instance *)
		ELSIF eControl_IEDLD1_LLN0_urcb101 <> E_AcsiCtlReport.None THEN
			IF eControl_IEDLD1_LLN0_urcb101 = E_AcsiCtlReport.Enable THEN (* Example => enable reporting *)
				
				(*
					Changing default properties of "Client" function block configures reporting behaviour and content of report message data.
					The "Client" function block writes the new property values to the server and enables RCB.
					In this example we use configuration values that were defined in the TwinCAT Telecontrol Configurator to control "urcb101".
				*)
				
				(* Configures "RptID" (report ID) to be used in report message *)
				fbIED.IEDLD1.LLN0.urcb101.Client.sRptID:= fbIED.IEDLD1.LLN0.urcb101.RptID.sConfig;(* => "IEDLD1/.LLN0.urcb101" *)
				
				(* Configures "TrgOps" (trigger options) to be used to trigger new report messages *)
				fbIED.IEDLD1.LLN0.urcb101.Client.cTrgOps:= fbIED.IEDLD1.LLN0.urcb101.TrgOps.cConfig;(* => All enabled except "DataUpdate" *)
				
				(* Configures "OptFlds" (optional fields) to be used in report message *)
				fbIED.IEDLD1.LLN0.urcb101.Client.cOptFlds:= fbIED.IEDLD1.LLN0.urcb101.OptFlds.cConfig;(* => All enabled except "BufferOverflow" and "EntryID" *)
				
				(* Configures "IntgPd" (period in milliseconds used to generate integrity report) *)
				fbIED.IEDLD1.LLN0.urcb101.Client.nIntgPd:= fbIED.IEDLD1.LLN0.urcb101.IntgPd.nConfig;(* => 2000ms *)
				
				(* Configures "BufTm" (max. report message buffer time in milliseconds) *)
				fbIED.IEDLD1.LLN0.urcb101.Client.nBufTm:= fbIED.IEDLD1.LLN0.urcb101.BufTm.nConfig;(* => 0ms *)
				
				(* Write properties and enable RCB *)
				bSuccess:= fbIED.IEDLD1.LLN0.urcb101.Client.EnableReq(ipClient:=fbConnection, ipDataSet:=fbIED.IEDLD1.LLN0.DS1, ipResult=>ipResult); (* Activation of command execution *)
				state:= SEL(bSuccess, 100, 11); (* If command activation succeeded then wait for command completion else report an error *)
			ELSIF eControl_IEDLD1_LLN0_urcb101 = E_AcsiCtlReport.Disable THEN (* Example => disable reporting *)
				bSuccess:= fbIED.IEDLD1.LLN0.urcb101.Client.DisableReq(ipResult=>ipResult); (* Activation of command execution *)
				state:= SEL(bSuccess, 100, 11); (* If command activation succeeded then wait for command completion else report an error *)
			ELSIF eControl_IEDLD1_LLN0_urcb101 = E_AcsiCtlReport.GI THEN (* Example => execute general interrogation *)
				bSuccess:= fbIED.IEDLD1.LLN0.urcb101.Client.GIReq(ipResult=>ipResult); (* Activation of command execution *)
				state:= SEL(bSuccess, 100, 11); (* If command activation succeeded then wait for command completion else report an error *)
			END_IF
			eControl_IEDLD1_LLN0_urcb101:= E_AcsiCtlReport.None; (* Reset enum value to recognize next write request *)
			
		(*==================================================================================================================================================================*)
		(* Control unbuffered reports using "IEDLD1/LLN0.urcb201.Client" function block instance *)
		ELSIF eControl_IEDLD1_LLN0_urcb201 <> E_AcsiCtlReport.None THEN
			IF eControl_IEDLD1_LLN0_urcb201 = E_AcsiCtlReport.Enable THEN (* Example => enable reporting *)
				(*
					Changing default properties of "Client" function block configures reporting behaviour and content of report message data (optional).
					The "Client" function block writes the new property values to the server and enables RCB.
					In this example we use the standard configuration values ​​of the function block "Client" to control the "urcb201":
					"fbIED.IEDLD1.LLN0.urcb201.Client.sRptID":= Empty string. Property "sRptID" is written if <> '' and differs from server value.
					"fbIED.IEDLD1.LLN0.urcb201.Client.cTrgOps":= All trigger options are enabled
					"fbIED.IEDLD1.LLN0.urcb201.Client.cOptFlds":= All options are enabled except "DataReference", "BufferOverflow" and "EntryID"
					"fbIED.IEDLD1.LLN0.urcb201.Client.nIntgPd":= Set to 5000ms
					"fbIED.IEDLD1.LLN0.urcb201.Client.nBufTm":= Set to 0ms
				*)
				(* Write properties and enable RCB *)
				bSuccess:= fbIED.IEDLD1.LLN0.urcb201.Client.EnableReq(ipClient:=fbConnection, ipDataSet:=fbIED.IEDLD1.LLN0.DS2, ipResult=>ipResult); (* Activation of command execution *)
				state:= SEL(bSuccess, 100, 11); (* If command activation succeeded then wait for command completion else report an error *)
			ELSIF eControl_IEDLD1_LLN0_urcb201 = E_AcsiCtlReport.Disable THEN (* Example => disable reporting *)
				bSuccess:= fbIED.IEDLD1.LLN0.urcb201.Client.DisableReq(ipResult=>ipResult); (* Activation of command execution *)
				state:= SEL(bSuccess, 100, 11); (* If command activation succeeded then wait for command completion else report an error *)
			ELSIF eControl_IEDLD1_LLN0_urcb201 = E_AcsiCtlReport.GI THEN (* Example => execute general interrogation *)
				bSuccess:= fbIED.IEDLD1.LLN0.urcb201.Client.GIReq(ipResult=>ipResult); (* Activation of command execution *)
				state:= SEL(bSuccess, 100, 11); (* If command activation succeeded then wait for command completion else report an error *)
			END_IF
			eControl_IEDLD1_LLN0_urcb201:= E_AcsiCtlReport.None; (* Reset enum value to recognize next write request *)

		(*==================================================================================================================================================================*)
		(* Control unbuffered reports using "IEDLD1/LLN0.urcb301.Client" function block instance *)
		ELSIF eControl_IEDLD1_LLN0_urcb301 <> E_AcsiCtlReport.None THEN
			IF eControl_IEDLD1_LLN0_urcb301 = E_AcsiCtlReport.Enable THEN (* Example => enable reporting *)
				
				(*
					Changing default properties of "Client" function block configures reporting behaviour and content of report message data.
					The "Client" function block writes the new property values to the server and enables RCB.
					In this example we use configuration values that were defined by application/user to control the "urcb301".
				*)
				
				(* Configures "RptID" (report ID) to be used in report message *)
				fbIED.IEDLD1.LLN0.urcb301.Client.sRptID:= 'IEDLD1/LLN0.RP.urcb301';
				
				(* Configures "TrgOps" (trigger options) to be used to trigger new report messages *)
				usrTrgOps.DataChange:= TRUE;
				usrTrgOps.DataUpdate:= FALSE;
				usrTrgOps.QualityChange:= FALSE;
				usrTrgOps.Integrity:= TRUE;
				usrTrgOps.GeneralInterrogation:= TRUE;
				fbIED.IEDLD1.LLN0.urcb301.Client.cTrgOps:= usrTrgOps;
				
				(* Configures "OptFlds" (option fields) to be used in report message *)
				usrOptFlds.ConfRevision:= TRUE;
				usrOptFlds.DataReference:= FALSE;
				usrOptFlds.DataSetName:= FALSE;
				usrOptFlds.ReasonForInclusion:= TRUE;
				usrOptFlds.ReportTimeStamp:= FALSE;
				usrOptFlds.SequenceNumber:= TRUE;
				usrOptFlds.BufferOverflow:= FALSE;
				usrOptFlds.EntryID:= FALSE;
				fbIED.IEDLD1.LLN0.urcb301.Client.cOptFlds:= usrOptFlds;
				
				(* Configures "IntgPd" (period in milliseconds used to generate integrity report) *)
				fbIED.IEDLD1.LLN0.urcb301.Client.nIntgPd:= 1000;
				
				(* Configures "BufTm" (max. report message buffer time in milliseconds) *)
				fbIED.IEDLD1.LLN0.urcb301.Client.nBufTm:= 500;
				
				(* Write properties and enable RCB *)
				bSuccess:= fbIED.IEDLD1.LLN0.urcb301.Client.EnableReq(ipClient:=fbConnection, ipDataSet:=fbIED.IEDLD1.LLN0.DS3, ipResult=>ipResult); (* Activation of command execution *)
				state:= SEL(bSuccess, 100, 11); (* If command activation succeeded then wait for command completion else report an error *)
			ELSIF eControl_IEDLD1_LLN0_urcb301 = E_AcsiCtlReport.Disable THEN (* Example => disable reporting *)
				bSuccess:= fbIED.IEDLD1.LLN0.urcb301.Client.DisableReq(ipResult=>ipResult); (* Activation of command execution *)
				state:= SEL(bSuccess, 100, 11); (* If command activation succeeded then wait for command completion else report an error *)
			ELSIF eControl_IEDLD1_LLN0_urcb301 = E_AcsiCtlReport.GI THEN (* Example => execute general interrogation *)
				bSuccess:= fbIED.IEDLD1.LLN0.urcb301.Client.GIReq(ipResult=>ipResult); (* Activation of command execution *)
				state:= SEL(bSuccess, 100, 11); (* If command activation succeeded then wait for command completion else report an error *)
			END_IF
			eControl_IEDLD1_LLN0_urcb301:= E_AcsiCtlReport.None; (* Reset enum value to recognize next write request *)
			
		(*==================================================================================================================================================================*)
		(* Control buffered reports using "IEDLD1/LLN0.brcb101.Client" function block instance *)
		ELSIF eControl_IEDLD1_LLN0_brcb101 <> E_AcsiCtlReport.None THEN
			IF eControl_IEDLD1_LLN0_brcb101 = E_AcsiCtlReport.Enable THEN (* Example => enable reporting using *)
				(*
					Changing default properties of "Client" function block configures reporting behaviour and content of report message data.
					The "Client" function block writes the new property values to the server and enables RCB.
					In this example we use configuration values that were defined in the TwinCAT Telecontrol Configurator to control "brcb101".
				*)
				
				(* Configures "RptID" to be used in report message *)
				fbIED.IEDLD1.LLN0.brcb101.Client.sRptID:= fbIED.IEDLD1.LLN0.brcb101.RptID.sConfig;(* => "IEDLD1/LLN0.brcb101" *)
				
				(* Configures "TrgOps" (trigger options) to be used to trigger new report messages *)
				fbIED.IEDLD1.LLN0.brcb101.Client.cTrgOps:= fbIED.IEDLD1.LLN0.brcb101.TrgOps.cConfig;(* => All enabled except "DataUpdate" *)
				
				(* Configures "OptFlds" (option fields) to be used in report message *)
				fbIED.IEDLD1.LLN0.brcb101.Client.cOptFlds:= fbIED.IEDLD1.LLN0.brcb101.OptFlds.cConfig;(* => All enabled *)
				
				(* Configures "IntgPd" (period in milliseconds used to generate integrity report) *)
				fbIED.IEDLD1.LLN0.brcb101.Client.nIntgPd:= fbIED.IEDLD1.LLN0.brcb101.IntgPd.nConfig;(* => 2000ms *)
				
				(* Configures "BufTm" (max. report message buffer time in milliseconds) *)
				fbIED.IEDLD1.LLN0.brcb101.Client.nBufTm:= fbIED.IEDLD1.LLN0.brcb101.BufTm.nConfig;(* => 0ms *)
				
				(* Write properties and enable RCB *)
				bSuccess:= fbIED.IEDLD1.LLN0.brcb101.Client.EnableReq(ipClient:=fbConnection, ipDataSet:=fbIED.IEDLD1.LLN0.DS1, ipResult=>ipResult); (* Activation of command execution *)
				state:= SEL(bSuccess, 100, 11); (* If command activation succeeded then wait for command completion else report an error *)
			ELSIF eControl_IEDLD1_LLN0_brcb101 = E_AcsiCtlReport.Disable THEN (* Example => disable reporting *)
				bSuccess:= fbIED.IEDLD1.LLN0.brcb101.Client.DisableReq(ipResult=>ipResult); (* Activation of command execution *)
				state:= SEL(bSuccess, 100, 11); (* If command activation succeeded then wait for command completion else report an error *)
			ELSIF eControl_IEDLD1_LLN0_brcb101 = E_AcsiCtlReport.GI THEN (* Example => execute general interrogation *)
				bSuccess:= fbIED.IEDLD1.LLN0.brcb101.Client.GIreq(ipResult=>ipResult); (* Activation of command execution *)
				state:= SEL(bSuccess, 100, 11); (* If command activation succeeded then wait for command completion else report an error *)
			ELSIF eControl_IEDLD1_LLN0_brcb101 = E_AcsiCtlReport.PurgeBuf THEN (* Example => execute purge buffer *)
				bSuccess:= fbIED.IEDLD1.LLN0.brcb101.Client.PurgeBufReq(ipClient:=fbConnection, ipResult=>ipResult); (* Activation of command execution *)
				state:= SEL(bSuccess, 100, 11); (* If command activation succeeded then wait for command completion else report an error *)
			ELSIF eControl_IEDLD1_LLN0_brcb101 = E_AcsiCtlReport.Resync THEN (* Example => execute resync *)
				bSuccess:= fbIED.IEDLD1.LLN0.brcb101.Client.ResyncReq(ipClient:=fbConnection, nEntryID:=Last_Rx_brcb101_nEntryID, ipResult=>ipResult); (* Activation of command execution *)
				state:= SEL(bSuccess, 100, 11); (* If command activation succeeded then wait for command completion else report an error *)
			END_IF
			eControl_IEDLD1_LLN0_brcb101:= E_AcsiCtlReport.None;(* Reset enum value to recognize next write request *)

		(*==================================================================================================================================================================*)
		(* Control buffered reports using "IEDLD1/LLN0.brcb201.Client" function block instance *)
		ELSIF eControl_IEDLD1_LLN0_brcb201 <> E_AcsiCtlReport.None THEN
			IF eControl_IEDLD1_LLN0_brcb201 = E_AcsiCtlReport.Enable THEN (* Example => enable reporting *)
				
				(*
					Changing default properties of "Client" function block configures reporting behaviour and content of report message data (optional).
					The "Client" function block writes the new property values to the server and enables RCB.
					In this example we use the standard configuration values ​​of the function block "Client" to control the "brcb201":
					"fbIED.IEDLD1.LLN0.brcb201.Client.sRptID":= Empty string. Property "sRptID" is only written if <> '' and differs from server value
					"fbIED.IEDLD1.LLN0.brcb201.Client.cTrgOps":= All trigger options are enabled
					"fbIED.IEDLD1.LLN0.brcb201.Client.cOptFlds":= All options are enabled except "DataReference"
					"fbIED.IEDLD1.LLN0.brcb201.Client.nIntgPd":= Set to 5000ms
					"fbIED.IEDLD1.LLN0.brcb201.Client.nBufTm":= Set to 0ms
				*)
				
				(* Write properties and enable RCB *)
				bSuccess:= fbIED.IEDLD1.LLN0.brcb201.Client.EnableReq(ipClient:=fbConnection, ipDataSet:=fbIED.IEDLD1.LLN0.DS2, ipResult=>ipResult); (* Activation of command execution *)
				state:= SEL(bSuccess, 100, 11); (* If command activation succeeded then wait for command completion else report an error *)
			ELSIF eControl_IEDLD1_LLN0_brcb201 = E_AcsiCtlReport.Disable THEN (* Example => disable reporting *)
				bSuccess:= fbIED.IEDLD1.LLN0.brcb201.Client.DisableReq(ipResult=>ipResult); (* Activation of command execution *)
				state:= SEL(bSuccess, 100, 11); (* If command activation succeeded then wait for command completion else report an error *)
			ELSIF eControl_IEDLD1_LLN0_brcb201 = E_AcsiCtlReport.GI THEN (* Example => execute general interrogation *)
				bSuccess:= fbIED.IEDLD1.LLN0.brcb201.Client.GIreq(ipResult=>ipResult); (* Activation of command execution *)
				state:= SEL(bSuccess, 100, 11); (* If command activation succeeded then wait for command completion else report an error *)
			ELSIF eControl_IEDLD1_LLN0_brcb201 = E_AcsiCtlReport.PurgeBuf THEN (* Example => execute purge buffer *)
				bSuccess:= fbIED.IEDLD1.LLN0.brcb201.Client.PurgeBufReq(ipClient:=fbConnection, ipResult=>ipResult); (* Activation of command execution *)
				state:= SEL(bSuccess, 100, 11); (* If command activation succeeded then wait for command completion else report an error *)
			ELSIF eControl_IEDLD1_LLN0_brcb201 = E_AcsiCtlReport.Resync THEN (* Example => execute resync *)
				bSuccess:= fbIED.IEDLD1.LLN0.brcb201.Client.ResyncReq(ipClient:=fbConnection, nEntryID:=Last_Rx_brcb201_nEntryID, ipResult=>ipResult); (* Activation of command execution *)
				state:= SEL(bSuccess, 100, 11); (* If command activation succeeded then wait for command completion else report an error *)
			END_IF
			eControl_IEDLD1_LLN0_brcb201:= E_AcsiCtlReport.None; (* Reset enum value to recognize next write request *)

		(*==================================================================================================================================================================*)
		(* Control buffered reports using "IEDLD1/LLN0.brcb301.Client" function block instance *)
		ELSIF eControl_IEDLD1_LLN0_brcb301 <> E_AcsiCtlReport.None THEN
			IF eControl_IEDLD1_LLN0_brcb301 = E_AcsiCtlReport.Enable THEN (* Example => enable reporting using *)
				
				(*
					Changing default properties of "Client" function block configures reporting behaviour and content of report message data.
					The "Client" function block writes the new property values to the server and enables RCB.
					In this example we use configuration values that were defined by application/user to control the "brcb301".
				*)
				
				(* Configures "RptID" (report ID) to be used in report message *)
				fbIED.IEDLD1.LLN0.brcb301.Client.sRptID:= 'IEDLD1/LLN0.BR.brcb301';
				
				(* Configures "TrgOps" (trigger options) to be used to trigger new report messages *)
				usrTrgOps.DataChange:= TRUE;
				usrTrgOps.DataUpdate:= FALSE;
				usrTrgOps.QualityChange:= FALSE;
				usrTrgOps.Integrity:= TRUE;
				usrTrgOps.GeneralInterrogation:= TRUE;
				fbIED.IEDLD1.LLN0.brcb301.Client.cTrgOps:= usrTrgOps;
				
				(* Configures "OptFlds" (option fields) to be used in report message *)
				usrOptFlds.ConfRevision:= TRUE;
				usrOptFlds.DataReference:= FALSE;
				usrOptFlds.DataSetName:= FALSE;
				usrOptFlds.ReasonForInclusion:= TRUE;
				usrOptFlds.ReportTimeStamp:= FALSE;
				usrOptFlds.SequenceNumber:= TRUE;
				usrOptFlds.BufferOverflow:= TRUE;
				usrOptFlds.EntryID:= TRUE;
				fbIED.IEDLD1.LLN0.brcb301.Client.cOptFlds:= usrOptFlds;

				(* Configures "IntgPd" (period in milliseconds used to generate integrity report) *)
				fbIED.IEDLD1.LLN0.brcb301.Client.nIntgPd:= 10000;

				(* Configures "BufTm" (max. report message buffer time in milliseconds) *)
				fbIED.IEDLD1.LLN0.brcb301.Client.nBufTm:= 500;

				(* Write properties and enable RCB *)
				bSuccess:= fbIED.IEDLD1.LLN0.brcb301.Client.EnableReq(ipClient:=fbConnection, ipDataSet:=fbIED.IEDLD1.LLN0.DS3, ipResult=>ipResult); (* Activation of command execution *)
				state:= SEL(bSuccess, 100, 11); (* If command activation succeeded then wait for command completion else report an error *)
			ELSIF eControl_IEDLD1_LLN0_brcb301 = E_AcsiCtlReport.Disable THEN (* Example => disable reporting *)
				bSuccess:= fbIED.IEDLD1.LLN0.brcb301.Client.DisableReq(ipResult=>ipResult); (* Activation of command execution *)
				state:= SEL(bSuccess, 100, 11); (* If command activation succeeded then wait for command completion else report an error *)
			ELSIF eControl_IEDLD1_LLN0_brcb301 = E_AcsiCtlReport.GI THEN (* Example => execute general interrogation *)
				bSuccess:= fbIED.IEDLD1.LLN0.brcb301.Client.GIreq(ipResult=>ipResult); (* Activation of command execution *)
				state:= SEL(bSuccess, 100, 11); (* If command activation succeeded then wait for command completion else report an error *)
			ELSIF eControl_IEDLD1_LLN0_brcb301 = E_AcsiCtlReport.PurgeBuf THEN (* Example => execute purge buffer *)
				bSuccess:= fbIED.IEDLD1.LLN0.brcb301.Client.PurgeBufReq(ipClient:=fbConnection, ipResult=>ipResult); (* Activation of command execution *)
				state:= SEL(bSuccess, 100, 11); (* If command activation succeeded then wait for command completion else report an error *)
			ELSIF eControl_IEDLD1_LLN0_brcb301 = E_AcsiCtlReport.Resync THEN (* Example => execute resync *)
				bSuccess:= fbIED.IEDLD1.LLN0.brcb301.Client.ResyncReq(ipClient:=fbConnection, nEntryID:=Last_Rx_brcb301_nEntryID, ipResult=>ipResult); (* Activation of command execution *)
				state:= SEL(bSuccess, 100, 11); (* If command activation succeeded then wait for command completion else report an error *)
			END_IF
			eControl_IEDLD1_LLN0_brcb301:= E_AcsiCtlReport.None; (* Reset enum value to recognize next write request *)
		ELSE
			state:= 0;
		END_IF
		(*==================================================================================================================================================================*)
	11: (* Wait for GetServerDirectoryReq(), GetLogicalDeviceDirectoryReq(), GetLogicalNodeDirectoryReq(), GetAllServerValuesReq(), GetAllDataValuesReq(), GetDataValuesReq(),
			GetUrCBValuesReq(), GetBrCBValuesReq(), SetUrCBValuesReq(), SetBrCBValuesReq() or report Enable/Disable/GI... command completion *)
		IF ipResult <> 0 THEN
			ipResult.Execute();
			IF NOT (bBusy:=ipResult.IsBusy()) THEN
				state:= SEL(ipResult.IsCompleted(), 100(* failed or aborted *), 0(* succeeded *));
			END_IF
		END_IF
		(*==================================================================================================================================================================*)
	100: (* Error state *)
		state:= 0;
		IF ipResult <> 0 THEN
			nCmdError:= nCmdError + 1;
			sLastErrorResult:= ipResult.Dump();
			fbIED.IEDLD1.LLN0.urcb101.client.Clear(ipReason:=ipResult.ipError);
			fbIED.IEDLD1.LLN0.brcb101.client.Clear(ipReason:=ipResult.ipError);
		END_IF
END_CASE

PROPERTY bAbort : BOOL
SET
_bAbort:= bAbort;
END_SET
END_PROPERTY

PROPERTY bConnect : BOOL
SET
_bConnect:= bConnect;
END_SET
END_PROPERTY

PROPERTY bDisconnect : BOOL
SET
_bDisconnect:= bDisconnect;
END_SET
END_PROPERTY

PROPERTY bReconnect : BOOL
SET
_bReconnect:= bReconnect;
END_SET
END_PROPERTY

(* This method receives IEC61850::Abort.ind primitive. *)
METHOD OnAbortInd
VAR_INPUT
	ipAA		: I_ScsmAssociationClass; (* Application association. If = 0 => optional. *)
	bPAbort		: BOOL; (* TRUE => P-Abort.request(), issued by provider, FALSE => Abort.request(), issued by user. *)
	ipReason	: I_ServiceErrorClass; (* Abort reason. *)
	ipData		: I_BaseStreamClass; (* Optional data. If = 0 => default, no data. *)
END_VAR
VAR
END_VAR
IF ipReason <> 0 THEN
	sLastAbortReason:= ipReason.Dump();
END_IF
END_METHOD

(* This method receives buffered IEC61850::Report.ind primitive. *)
METHOD OnBufferedReportInd
VAR_INPUT
	ipAA		: I_ScsmAssociationClass; (* Application association. If = 0 => optional. *)
	info		: ST_ScsmReportEventInfo;
	ipBrcb		: I_AcsiCommonBufferedReportControlBlockClass; (* Interface pointer to BRCB object. *)
	ipDataSet	: I_AcsiCommonDataSetClass; (* Interface pointer to data-set object. *)
	ipData		: I_AcsiCommonDataClass; (* Interface pointer to reported data object. *)
	eFc			: E_AcsiFc; (* Functional constraint of reported data. *)
	eError		: E_AcsiServiceError; (* Data access error code. *)
END_VAR
VAR
	sBrcbRef	: T_AcsiObjectReference;
END_VAR
IF eError <> E_AcsiServiceError.NoError THEN
	eServiceError:= eError;
	nServiceError:= nServiceError + 1;
END_IF
IF ipData <> 0 THEN
	sObjReference:= ipData.GetObjectReference();
END_IF
IF ipBrcb <> 0 THEN
	sBrcbRef:=ipBrcb.GetObjectReference();
	IF sBrcbRef = 'IEDLD1/LLN0.brcb101' THEN
		Last_Rx_brcb101_nEntryID := AcsiEntryID_To_LWORD(info.EntryID, TRUE);
	ELSIF sBrcbRef = 'IEDLD1/LLN0.brcb201' THEN
		Last_Rx_brcb201_nEntryID := AcsiEntryID_To_LWORD(info.EntryID, TRUE);
	ELSIF sBrcbRef = 'IEDLD1/LLN0.brcb301' THEN
		Last_Rx_brcb301_nEntryID := AcsiEntryID_To_LWORD(info.EntryID, TRUE);
	END_IF
END_IF
END_METHOD

(* This method receives IEC61850::CommandTermination.ind primitive. *)
METHOD OnCommandTerminationInd
VAR_INPUT
	ipAA		: I_ScsmAssociationClass; (* Application association. If = 0 => optional. *)
	info		: ST_ScsmCommandTerminationEventInfo;
	ipCtrl		: I_AcsiCommonControllableDataClass; (* Interface pointer to controllable data object. *)
	ipData		: I_AcsiCommonDataClass; (* Interface pointer to Oper/Cancel/SBO or SBOw data object. *)
	eFc			: E_AcsiFc; (* Functional constraint (CO). *)
	eError		: E_AcsiServiceError; (* Error code. *)
END_VAR
VAR
END_VAR
IF eError <> E_AcsiServiceError.NoError THEN
	eServiceError:= eError;
	nServiceError:= nServiceError + 1;
END_IF
IF ipCtrl <> 0 THEN
	sCtrlReference:= ipCtrl.GetObjectReference();
END_IF
IF ipData <> 0 THEN
	sObjReference:= ipData.GetObjectReference();
END_IF
END_METHOD

(* This method receives IEC61850::Control[Select|Operate|SelectWithValue|Cancel].cnf primitive. *)
METHOD OnControlCnf
VAR_INPUT
	ipAA		: I_ScsmAssociationClass; (* Application association. If = 0 => optional. *)
	info		: ST_ScsmConfirmedEventInfo;
	ipCtrl		: I_AcsiCommonControllableDataClass; (* Interface pointer to controllable data object. *)
	ipData		: I_AcsiCommonDataClass; (* Interface pointer to Oper/Cancel/SBO or SBOw data object. *)
	eFc			: E_AcsiFc; (* Functional constraint (CO). *)
	eError		: E_AcsiServiceError; (* Write/Read data access error code. *)
END_VAR
VAR
END_VAR
IF eError <> E_AcsiServiceError.NoError THEN
	eServiceError:= eError;
	nServiceError:= nServiceError + 1;
END_IF
IF ipCtrl <> 0 THEN
	sCtrlReference:= ipCtrl.GetObjectReference();
END_IF
IF ipData <> 0 THEN
	sObjReference:= ipData.GetObjectReference();
END_IF
END_METHOD

(* This method receives IEC61850::GetDataValues.cnf primitive. *)
METHOD OnGetDataValuesCnf
VAR_INPUT
	ipAA		: I_ScsmAssociationClass; (* Application association. If = 0 => optional. *)
	info		: ST_ScsmConfirmedEventInfo;
	ipData		: I_AcsiCommonDataClass; (* Interface pointer to read data object. *)
	eFc			: E_AcsiFc; (* Functional constraint of read data. *)
	eError		: E_AcsiServiceError; (* Data access error code. *)
END_VAR
VAR
END_VAR
IF eError <> E_AcsiServiceError.NoError THEN
	eServiceError:= eError;
	nServiceError:= nServiceError + 1;
END_IF
IF ipData <> 0 THEN
	sObjReference:= ipData.GetObjectReference();
END_IF
END_METHOD

(* This method receives IEC61850::GetLogicalDeviceDirectory.cnf primitive. *)
METHOD OnGetLogicalDeviceDirectoryCnf
VAR_INPUT
	ipAA				: I_ScsmAssociationClass; (* Application association. If = 0 => optional. *)
	info				: ST_ScsmConfirmedEventInfo;
	ipLogicalDevice		: I_AcsiCommonLogicalDeviceClass; (* Interface pointer to logical-device object. *)
	sObjectReference	: T_AcsiObjectReference;
	eError				: E_AcsiServiceError; (* Logical-device class access error code. *)
END_VAR
VAR
END_VAR
IF eError <> E_AcsiServiceError.NoError THEN
	eServiceError:= eError;
	nServiceError:= nServiceError + 1;
END_IF
sObjReference:= sObjectReference;
END_METHOD

(* This method receives IEC61850::GetLogicalNodeDirectory.cnf primitive. *)
METHOD OnGetLogicalNodeDirectoryCnf
VAR_INPUT
	ipAA				: I_ScsmAssociationClass; (* Application association. If = 0 => optional. *)
	info				: ST_ScsmConfirmedEventInfo;
	ipLogicalNode		: I_AcsiCommonLogicalNodeClass; (* Interface pointer to logical-node object. *)
	eClass				: E_AcsiLogicalNodeClass; (* Logical-node directory class (BRCB, URCB, DATA-SET, ... ). *)
	sObjectReference	: T_AcsiObjectReference;
	eError				: E_AcsiServiceError; (* Logical-node class access error code. *)
END_VAR
VAR
END_VAR
IF eError <> E_AcsiServiceError.NoError THEN
	eServiceError:= eError;
	nServiceError:= nServiceError + 1;
END_IF
sObjReference:= sObjectReference;
END_METHOD

(* This method receives IEC61850::GetServerDirectory.cnf primitive. *)
METHOD OnGetServerDirectoryCnf
VAR_INPUT
	ipAA				: I_ScsmAssociationClass; (* Application association. If = 0 => optional. *)
	info				: ST_ScsmConfirmedEventInfo;
	ipServer			: I_AcsiCommonIntelligentElectronicDeviceClass; (* Interface pointer to server object. *)
	eClass				: E_AcsiServerDirectoryClass; (* Server directory class (logical-device or file). *)
	sObjectReference	: T_AcsiObjectReference;
	eError				: E_AcsiServiceError; (* Server class (logical-device) access error code. *)
END_VAR
VAR
END_VAR
IF eError <> E_AcsiServiceError.NoError THEN
	eServiceError:= eError;
	nServiceError:= nServiceError + 1;
END_IF
sObjReference:= sObjectReference;
END_METHOD

(* This method receives IEC61850::LastApplError.ind primitive. *)
METHOD OnLastApplErrorInd
VAR_INPUT
	ipAA		: I_ScsmAssociationClass; (* Application association. If = 0 => optional. *)
	info		: ST_ScsmAdditionalCauseDiagnosticEventInfo;
	ipCtrl		: I_AcsiCommonControllableDataClass; (* Interface pointer to controllable data object. *)
	eError		: E_AcsiServiceError; (* Error code. *)
END_VAR
VAR
END_VAR
IF eError <> E_AcsiServiceError.NoError THEN
	eServiceError:= eError;
	nServiceError:= nServiceError + 1;
END_IF
IF ipCtrl <> 0 THEN
	sCtrlReference:= ipCtrl.GetObjectReference();
END_IF
END_METHOD

(* This method receives IEC61850::SetDataValues.cnf primitive. *)
METHOD OnSetDataValuesCnf
VAR_INPUT
	ipAA		: I_ScsmAssociationClass; (* Application association. If = 0 => optional. *)
	info		: ST_ScsmConfirmedEventInfo;
	ipData		: I_AcsiCommonDataClass; (* Interface pointer to written data object. *)
	eFc			: E_AcsiFc; (* Functional constraint of written data. *)
	eError		: E_AcsiServiceError; (* Data access error code. *)
END_VAR
VAR
END_VAR
IF eError <> E_AcsiServiceError.NoError THEN
	eServiceError:= eError;
	nServiceError:= nServiceError + 1;
END_IF
IF ipData <> 0 THEN
	sObjReference:= ipData.GetObjectReference();
END_IF
END_METHOD

(* This method receives unbuffered IEC61850::Report.ind primitive. *)
METHOD OnUnbufferedReportInd
VAR_INPUT
	ipAA		: I_ScsmAssociationClass; (* Application association. If = 0 => optional. *)
	info		: ST_ScsmReportEventInfo;
	ipUrcb		: I_AcsiCommonUnbufferedReportControlBlockClass; (* Interface pointer to URCB object. *)
	ipDataSet	: I_AcsiCommonDataSetClass; (* Interface pointer to dataset object. *)
	ipData		: I_AcsiCommonDataClass; (* Interface pointer to reported data object. *)
	eFc			: E_AcsiFc; (* Functional constraint of reported data. *)
	eError		: E_AcsiServiceError; (* Data access error code. *)
END_VAR
VAR
END_VAR
IF eError <> E_AcsiServiceError.NoError THEN
	eServiceError:= eError;
	nServiceError:= nServiceError + 1;
END_IF
IF ipData <> 0 THEN
	sObjReference:= ipData.GetObjectReference();
END_IF
END_METHOD

END_FUNCTION_BLOCK
